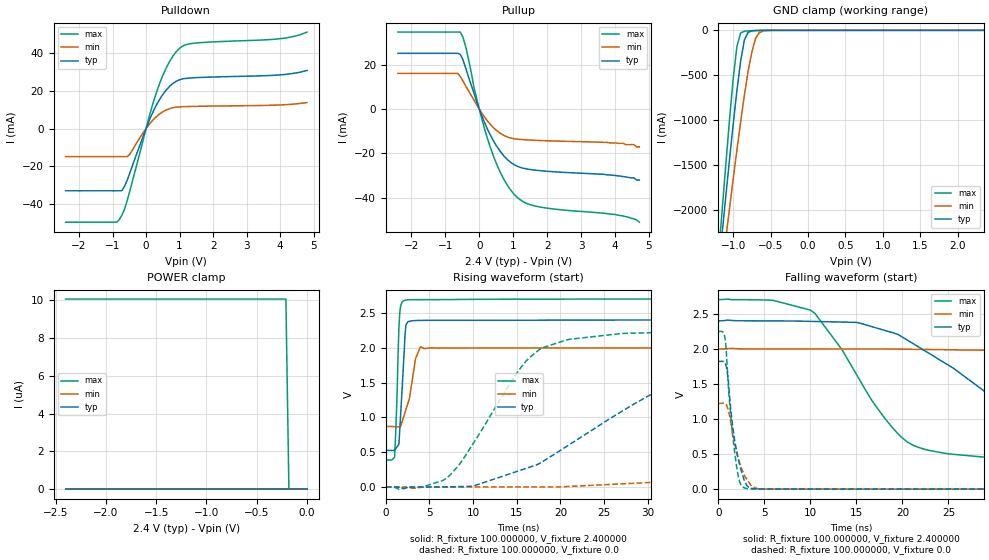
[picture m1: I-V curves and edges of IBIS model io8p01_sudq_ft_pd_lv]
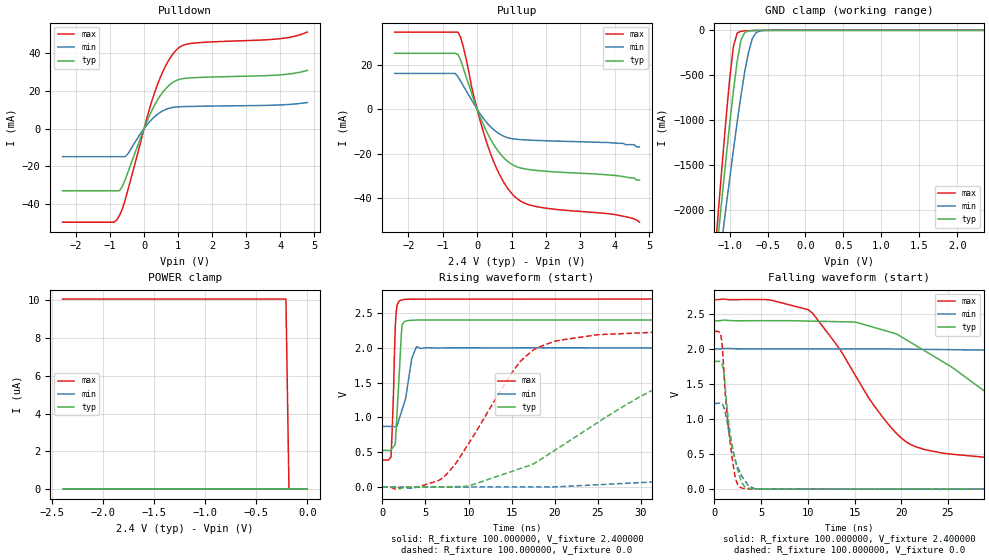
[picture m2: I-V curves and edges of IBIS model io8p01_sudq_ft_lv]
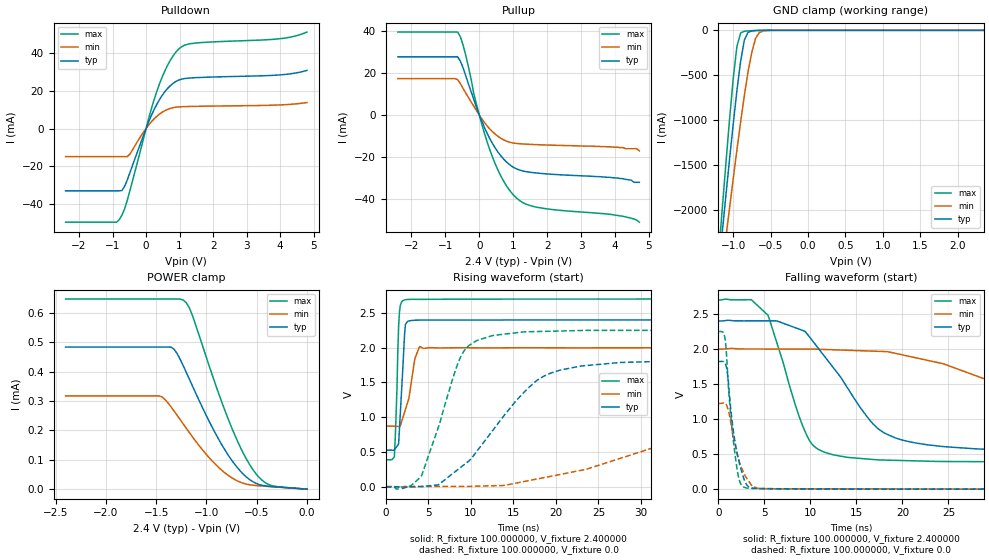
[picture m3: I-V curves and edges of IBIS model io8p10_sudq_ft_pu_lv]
|   stm32f0_444_tssop20 IBIS Model
[IBIS ver]   4.2
[File name]  stm32f0_444_tssop20.ibs
[File Rev]   1.0
[Date]   15-5-2013
[Source] Data Created at STMicroelectronics
[Notes]   File originated from ELDO simulations.
[Disclaimer]  This information is for modeling purpose only and is
   not guaranted. The information is subject to change without
   notice.
[Copyright] Copyright 2015 STMicroelectronics Inc.
[Component] stm32f0_444_tssop20
[Manufacturer] STMicroelectronics
[Package]
| variable   typ   min   max
R_pkg   0.0   NA   NA
L_pkg   0.0H   NA   NA
C_pkg   0.0F   NA   NA
[Pin] signal_name  model_name   R_pin   L_pin   C_pin
1   BOOT0 vpp_test_hv   23.0E-3   1.4E-9   40.0E-15
2   PF0   io8p_sudq_ft   18.1E-3   896.7E-12   15.0E-15
3   PF1   io8p_sudq_ft   16.4E-3   726.7E-12   6.7E-15
4   NRST  ioreset_tc_v33   18.1E-3   896.7E-12   15.0E-15
5   VDDA  POWER   23.0E-3   1.4E-9   40.0E-15
6   PA0   io8p_sudq_ft   23.0E-3   1.4E-9   40.0E-15
7   PA1   io8p_sudq_ft   18.1E-3   896.7E-12   15.0E-15
8   PA2   io8p_sudq_ft   16.4E-3   726.7E-12   6.7E-15
9   PA3   io8p_sudq_ft   18.1E-3   896.7E-12   15.0E-15
10   PA4   io8p_sudq_ft   23.0E-3   1.4E-9   40.0E-15
11   PA5   io8p_sudq_ft   23.0E-3   1.4E-9   40.0E-15
12   PA6   io8p_sudq_ft   18.1E-3   896.7E-12   15.0E-15
13   PA7   io8p_sudq_ft   16.4E-3   726.7E-12   6.7E-15
14   PB1   io8p_sudq_ft   18.1E-3   896.7E-12   15.0E-15
15   VSS   GND   23.0E-3   1.4E-9   40.0E-15
16   VDD   POWER   23.0E-3   1.4E-9   40.0E-15
17   PA9   io8p_sudq_ft   18.1E-3   896.7E-12   15.0E-15
18   PA10  io8p_sudq_ft   16.4E-3   726.7E-12   6.7E-15
19   PA13  io8p_sudq_ft   18.1E-3   896.7E-12   15.0E-15
20   PA14  io8p_sudq_ft   23.0E-3   1.4E-9   40.0E-15
[Model Selector] io8p_sudq_ft
io8p01_sudq_ft_pd_lv  "SPEED01 2P0V, PD=40kOhm"
io8p01_sudq_ft_pu_lv  "SPEED01 2P0V, PU=40kOhm"
io8p01_sudq_ft_lv  "SPEED01 2P0V"
io8p10_sudq_ft_pd_lv  "SPEED10 2P0V, PD=40kOhm"
io8p10_sudq_ft_pu_lv  "SPEED10 2P0V, PU=40kOhm"
io8p10_sudq_ft_lv  "SPEED10 2P0V"
io8p11_sudq_ft_pd_lv  "SPEED11 2P0V, PD=40kOhm"
io8p11_sudq_ft_pu_lv  "SPEED11 2P0V, PU=40kOhm"
io8p11_sudq_ft_lv  "SPEED11 2P0V"
io8p01_sudq_ft_pd  "SPEED01, PD=40kOhm"
io8p01_sudq_ft_pu  "SPEED01, PU=40kOhm"
io8p01_sudq_ft  "SPEED01"
io8p10_sudq_ft_pd  "SPEED10, PD=40kOhm"
io8p10_sudq_ft_pu  "SPEED10, PU=40kOhm"
io8p10_sudq_ft  "SPEED10"
io8p11_sudq_ft_pd  "SPEED11, PD=40kOhm"
io8p11_sudq_ft_pu  "SPEED11, PU=40kOhm"
io8p11_sudq_ft  "SPEED11"
[Model Selector] ioreset_tc_v33
ioreset_tc_v33_pu_lv  "IORESET 2V + PU=40kOhm"
ioreset_tc_v33_nopu_lv  "IORESET 2V"
ioreset_tc_v33_pu  "IORESET + PU=40kOhm"
ioreset_tc_v33_nopu  "IORESET"
[Model Selector] vpp_test_hv
vpp_test_hv_3p3  "Input Buffer"
vpp_test_hv_2p4  "Input Buffer 2P0V"
| Models and submodels in the file (24): io8p01_sudq_ft_pd_lv (I/O), io8p01_sudq_ft_pu_lv (I/O), io8p01_sudq_ft_lv (I/O), io8p10_sudq_ft_pd_lv (I/O), io8p10_sudq_ft_pu_lv (I/O), io8p10_sudq_ft_lv (I/O), io8p11_sudq_ft_pd_lv (I/O), io8p11_sudq_ft_pu_lv (I/O), io8p11_sudq_ft_lv (I/O), io8p01_sudq_ft_pd (I/O), io8p01_sudq_ft_pu (I/O), io8p01_sudq_ft (I/O), io8p10_sudq_ft_pd (I/O), io8p10_sudq_ft_pu (I/O), io8p10_sudq_ft (I/O), io8p11_sudq_ft_pd (I/O), io8p11_sudq_ft_pu (I/O), io8p11_sudq_ft (I/O), ioreset_tc_v33_pu_lv (I/O_open_drain), ioreset_tc_v33_nopu_lv (I/O_open_drain), ioreset_tc_v33_pu (I/O_open_drain), ioreset_tc_v33_nopu (I/O_open_drain), vpp_test_hv_2p4 (Input), vpp_test_hv_3p3 (Input)
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|   Model io8p01_sudq_ft_pd_lv
[Model]  io8p01_sudq_ft_pd_lv
Model_type I/O
Polarity   Non-Inverting
Enable   Active-Low
Vinl =   0.720000V
Vinh =   1.680000V
Vmeas =  1.200000V
Cref =   50.000000pF
Rref =   100.000000M
Vref =   0.0V
C_comp   1.970100pF   1.887900pF   2.069400pF
[Temperature Range]   25.000000   0.125000k   -40.000000
[Pullup Reference]   2.400000V   2.000000V   2.700000V
[Pulldown Reference]   0.0V   0.0V   0.0V
[POWER Clamp Reference]   2.400000V   2.000000V   2.700000V
[GND Clamp Reference]   0.0V   0.0V   0.0V
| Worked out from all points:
|   slope of the pulldown table from 0 to 0.36 V, typ, clamps not added: 25.5 ohm
|   slope of the pullup table from 0 to 0.36 V, typ, clamps not added: 28.4 ohm
|   GND clamp passes 1 mA (typ) near -0.64 V on its own axis
|   rising waveform, R_fixture 100.000000, V_fixture 2.400000: 20-80 % time 499ps typ, 1.06ns min, 336ps max; typ from 0.525 V to 2.4 V
|   rising waveform, R_fixture 100.000000, V_fixture 0.0: 20-80 % time 14.6ns typ, 43.7ns min, 6.88ns max; typ from 0 V to 1.82 V
|   falling waveform, R_fixture 100.000000, V_fixture 2.400000: 20-80 % time 12.9ns typ, 32.5ns min, 7.07ns max; typ from 2.4 V to 0.525 V
|   falling waveform, R_fixture 100.000000, V_fixture 0.0: 20-80 % time 1.15ns typ, 1.36ns min, 910ps max; typ from 1.82 V to 0 V
[Pulldown]
|Voltage   I(typ)   I(min)   I(max)
-2.4V     -33.16mA   -14.98mA   -49.86mA
-880mV    -33.16mA   -14.98mA   -49.86mA
-800mV    -33.16mA   -14.98mA   -48.55mA
-640mV    -30.75mA   -14.98mA   -42.76mA
-480mV    -23.43mA   -13.57mA   -32.92mA
80mV      3.651mA    1.905mA    5.506mA
400mV     15.37mA    7.665mA    23.73mA
720mV     22.75mA    10.69mA    36.23mA
1.04V     26.18mA    11.57mA    43.27mA
1.52V     27.09mA    11.81mA    45.55mA
4V        28.55mA    12.55mA    47.81mA
4.8V      30.9mA     13.81mA    51.31mA
[Pullup]
|Voltage   I(typ)   I(min)   I(max)
-2.4V     25.2mA     16.13mA    34.79mA
-640mV    25.2mA     16.13mA    34.79mA
-560mV    24.71mA    14.75mA    34.79mA
-400mV    18.51mA    10.48mA    28.09mA
-160mV    7.338mA    4.152mA    10.02mA
80mV      -3.229mA   -1.94mA    -4.736mA
400mV     -13.82mA   -8.081mA   -20.45mA
800mV     -22.31mA   -12.38mA   -33.66mA
1.2V      -26.24mA   -13.65mA   -40.83mA
1.76V     -27.69mA   -14.12mA   -44.07mA
4V        -29.9mA    -15.2mA    -47.5mA
4.72V     -32mA      -17mA      -51mA
[GND_clamp]
|Voltage   I(typ)   I(min)   I(max)
-2.4V     -9.788A    -9.782A    -9.734A
-1.2V     -2.718A    -3.021A    -2.568A
-1.15V    -2.29A     -2.675A    -2.036A
-1.1V     -1.868A    -2.333A    -1.515A
-1.05V    -1.454A    -1.995A    -1.012A
-950mV    -674.5mA   -1.337A    -180.6mA
-900mV    -345.2mA   -1.023A    -29.74mA
-850mV    -106.4mA   -726mA     -10.14mA
-750mV    -6.411mA   -244mA     -4.042mA
-700mV    -2.572mA   -88.62mA   -2.346mA
-600mV    -429.6uA   -7.75mA    -383.5uA
2.35V     59.77uA    46.33uA    66.89uA
[POWER_clamp]
|Voltage   I(typ)   I(min)   I(max)
-2.4V     0A         0A         10.06uA
-210mV    0A         0A         10.06uA
-180mV    0A         0A         0A
0V        0A         0A         0A
[Ramp]
| variable   typ   min   max
dV/dt_r  1.09218/14.55718n   0.73266/43.64565n   1.34874/6.87247n
dV/dt_f  1.12429/12.86053n   0.67801/32.45722n   1.38701/7.06387n
R_load = 100.000000
[Rising Waveform]
R_fixture= 100.000000
V_fixture= 2.400000
V_fixture_min= 2.000000
V_fixture_max= 2.700000
|time   V(typ)   V(min)   V(max)
0s        524.8mV    868.7mV    387.2mV
1.001ns   533mV      867mV      427.7mV
1.301ns   579.7mV    865.4mV    1.395V
1.502ns   618.4mV    864.7mV    2.307V
1.602ns   837.8mV    864.4mV    2.512V
2.102ns   1.961V     1.034V     2.677V
2.302ns   2.331V     1.113V     2.684V
3.403ns   2.39V      1.843V     2.691V
4.004ns   2.392V     2.014V     2.691V
49.85ns   2.399V     1.999V     2.699V
[Rising Waveform]
R_fixture= 100.000000
V_fixture= 0.0
V_fixture_min= 0.0
V_fixture_max= 0.0
|time   V(typ)   V(min)   V(max)
0s        1.768nV    15.89nV    1.355nV
7.007ns   1.867mV    822uV      130.1mV
15.02ns   222.8mV    610.6uV    1.635V
17.52ns   330.7mV    351.7uV    1.966V
27.03ns   1.085V     44.44mV    2.204V
34.53ns   1.55V      90.81mV    2.229V
43.04ns   1.723V     239mV      2.246V
84.08ns   1.82V      945.5mV    2.248V
103.1ns   1.82V      1.111V     2.248V
249.2ns   1.82V      1.221V     2.248V
[Falling Waveform]
R_fixture= 100.000000
V_fixture= 2.400000
V_fixture_min= 2.000000
V_fixture_max= 2.700000
|time   V(typ)   V(min)   V(max)
0s        2.399V     1.999V     2.699V
10.01ns   2.391V     1.998V     2.551V
15.02ns   2.376V     1.997V     1.633V
20.02ns   2.165V     1.994V     725.2mV
29.53ns   1.332V     1.979V     449.6mV
35.04ns   877.6mV    1.964V     425.1mV
42.54ns   673.2mV    1.851V     405.8mV
67.07ns   552.7mV    1.286V     389.2mV
85.59ns   536.1mV    1.035V     387.2mV
249.2ns   524.8mV    868.7mV    387.2mV
[Falling Waveform]
R_fixture= 100.000000
V_fixture= 0.0
V_fixture_min= 0.0
V_fixture_max= 0.0
|time   V(typ)   V(min)   V(max)
0s        1.82V      1.221V     2.248V
700.7ps   1.801V     1.221V     2.178V
800.8ps   1.783V     1.214V     2.095V
1.001ns   1.652V     1.164V     1.701V
1.401ns   1.088V     921.6mV    989mV
1.802ns   687.3mV    646.2mV    513.2mV
2.302ns   364.2mV    381.5mV    115.5mV
2.903ns   104.2mV    178.7mV    14.94mV
4.705ns   1.559mV    3.204mV    789.6uV
49.85ns   1.768nV    15.89nV    1.355nV
|   Model io8p01_sudq_ft_lv
[Model]  io8p01_sudq_ft_lv
Model_type I/O
Polarity   Non-Inverting
Enable   Active-Low
Vinl =   0.720000V
Vinh =   1.680000V
Vmeas =  1.200000V
Cref =   50.000000pF
Rref =   100.000000M
Vref =   0.0V
C_comp   1.970100pF   1.887900pF   2.069400pF
[Temperature Range]   25.000000   0.125000k   -40.000000
[Pullup Reference]   2.400000V   2.000000V   2.700000V
[Pulldown Reference]   0.0V   0.0V   0.0V
[POWER Clamp Reference]   2.400000V   2.000000V   2.700000V
[GND Clamp Reference]   0.0V   0.0V   0.0V
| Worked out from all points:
|   slope of the pulldown table from 0 to 0.36 V, typ, clamps not added: 25.5 ohm
|   slope of the pullup table from 0 to 0.36 V, typ, clamps not added: 28.4 ohm
|   GND clamp passes 1 mA (typ) near -0.64 V on its own axis
|   rising waveform, R_fixture 100.000000, V_fixture 2.400000: 20-80 % time 499ps typ, 1.06ns min, 336ps max; typ from 0.525 V to 2.4 V
|   rising waveform, R_fixture 100.000000, V_fixture 0.0: 20-80 % time 14.5ns typ, 43.7ns min, 6.87ns max; typ from 0 V to 1.82 V
|   falling waveform, R_fixture 100.000000, V_fixture 2.400000: 20-80 % time 13ns typ, 32.3ns min, 7.05ns max; typ from 2.4 V to 0.525 V
|   falling waveform, R_fixture 100.000000, V_fixture 0.0: 20-80 % time 1.16ns typ, 1.39ns min, 931ps max; typ from 1.82 V to 0 V
[Pulldown]
|Voltage   I(typ)   I(min)   I(max)
-2.4V     -33.16mA   -14.98mA   -49.86mA
-880mV    -33.16mA   -14.98mA   -49.86mA
-800mV    -33.16mA   -14.98mA   -48.55mA
-640mV    -30.75mA   -14.98mA   -42.76mA
-480mV    -23.43mA   -13.57mA   -32.92mA
80mV      3.651mA    1.905mA    5.506mA
400mV     15.37mA    7.665mA    23.73mA
720mV     22.75mA    10.69mA    36.23mA
1.04V     26.18mA    11.57mA    43.27mA
1.52V     27.09mA    11.81mA    45.55mA
4V        28.55mA    12.55mA    47.81mA
4.8V      30.9mA     13.81mA    51.31mA
[Pullup]
|Voltage   I(typ)   I(min)   I(max)
-2.4V     25.21mA    16.13mA    34.79mA
-640mV    25.21mA    16.13mA    34.79mA
-560mV    24.72mA    14.75mA    34.79mA
-400mV    18.51mA    10.48mA    28.09mA
-160mV    7.322mA    4.15mA     10.02mA
80mV      -3.229mA   -1.94mA    -4.736mA
400mV     -13.82mA   -8.081mA   -20.45mA
800mV     -22.31mA   -12.38mA   -33.66mA
1.2V      -26.24mA   -13.65mA   -40.83mA
1.76V     -27.69mA   -14.12mA   -44.07mA
4V        -29.9mA    -15.2mA    -47.5mA
4.72V     -32mA      -17mA      -51mA
[GND_clamp]
|Voltage   I(typ)   I(min)   I(max)
-2.4V     -9.788A    -9.782A    -9.734A
-1.2V     -2.718A    -3.02A     -2.568A
-1.15V    -2.29A     -2.675A    -2.036A
-1.1V     -1.868A    -2.333A    -1.515A
-1.05V    -1.454A    -1.995A    -1.012A
-950mV    -674.5mA   -1.337A    -180.5mA
-900mV    -345.2mA   -1.023A    -29.72mA
-850mV    -106.4mA   -726mA     -10.13mA
-750mV    -6.396mA   -244mA     -4.026mA
-700mV    -2.558mA   -88.61mA   -2.329mA
-600mV    -416uA     -7.739mA   -368uA
2.35V     0A         0A         0A
[POWER_clamp]
|Voltage   I(typ)   I(min)   I(max)
-2.4V     0A         0A         10.06uA
-210mV    0A         0A         10.06uA
-180mV    0A         0A         0A
0V        0A         0A         0A
[Ramp]
| variable   typ   min   max
dV/dt_r  1.09308/14.53591n   0.73368/43.60005n   1.34946/6.86189n
dV/dt_f  1.12469/12.94342n   0.67781/32.23620n   1.38756/7.04174n
R_load = 100.000000
[Rising Waveform]
R_fixture= 100.000000
V_fixture= 2.400000
V_fixture_min= 2.000000
V_fixture_max= 2.700000
|time   V(typ)   V(min)   V(max)
0s        525.2mV    870.3mV    387.4mV
1.001ns   533.4mV    868.6mV    427.9mV
1.301ns   580.2mV    867mV      1.396V
1.502ns   618.9mV    866.4mV    2.308V
1.702ns   1.058V     877.1mV    2.607V
2.202ns   2.2V       1.075V     2.686V
2.703ns   2.383V     1.274V     2.696V
3.403ns   2.395V     1.844V     2.698V
4.004ns   2.398V     2.016V     2.698V
49.85ns   2.4V       2V         2.7V
[Rising Waveform]
R_fixture= 100.000000
V_fixture= 0.0
V_fixture_min= 0.0
V_fixture_max= 0.0
|time   V(typ)   V(min)   V(max)
0s        1.81nV     16.19nV    1.388nV
7.007ns   1.867mV    817.4uV    130.2mV
16.52ns   286.2mV    456uV      1.866V
20.02ns   528mV      1.164mV    2.095V
25.03ns   931.2mV    32.13mV    2.189V
37.04ns   1.629V     132.6mV    2.24V
54.55ns   1.791V     444.2mV    2.251V
84.08ns   1.821V     947.3mV    2.249V
106.1ns   1.822V     1.128V     2.249V
249.2ns   1.822V     1.223V     2.249V
[Falling Waveform]
R_fixture= 100.000000
V_fixture= 2.400000
V_fixture_min= 2.000000
V_fixture_max= 2.700000
|time   V(typ)   V(min)   V(max)
0s        2.4V       2V         2.7V
10.01ns   2.397V     2V         2.56V
15.02ns   2.383V     2V         1.637V
20.02ns   2.171V     1.997V     726.6mV
29.03ns   1.387V     1.983V     453.9mV
37.04ns   789.8mV    1.94V      415.8mV
52.55ns   592.4mV    1.669V     394.5mV
72.57ns   546.2mV    1.209V     388.6mV
99.1ns    528mV      969.1mV    387.4mV
249.2ns   525.2mV    870.3mV    387.4mV
[Falling Waveform]
R_fixture= 100.000000
V_fixture= 0.0
V_fixture_min= 0.0
V_fixture_max= 0.0
|time   V(typ)   V(min)   V(max)
0s        1.822V     1.223V     2.249V
700.7ps   1.802V     1.223V     2.18V
800.8ps   1.785V     1.216V     2.097V
1.001ns   1.655V     1.166V     1.704V
1.201ns   1.378V     1.071V     1.289V
1.902ns   616.6mV    591.6mV    436.6mV
2.302ns   369.3mV    388.2mV    131.7mV
2.903ns   108.1mV    191.2mV    18.1mV
4.705ns   2.197mV    4.103mV    1.139mV
49.85ns   1.81nV     16.19nV    1.388nV
|   Model io8p10_sudq_ft_pu_lv
[Model]  io8p10_sudq_ft_pu_lv
Model_type I/O
Polarity   Non-Inverting
Enable   Active-Low
Vinl =   0.720000V
Vinh =   1.680000V
Vmeas =  1.200000V
Cref =   50.000000pF
Rref =   100.000000M
Vref =   0.0V
C_comp   1.970100pF   1.887900pF   2.069400pF
[Temperature Range]   25.000000   0.125000k   -40.000000
[Pullup Reference]   2.400000V   2.000000V   2.700000V
[Pulldown Reference]   0.0V   0.0V   0.0V
[POWER Clamp Reference]   2.400000V   2.000000V   2.700000V
[GND Clamp Reference]   0.0V   0.0V   0.0V
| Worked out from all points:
|   slope of the pulldown table from 0 to 0.36 V, typ, clamps not added: 25.5 ohm
|   slope of the pullup table from 0 to 0.36 V, typ, clamps not added: 28.4 ohm
|   GND clamp passes 1 mA (typ) near -0.64 V on its own axis
|   rising waveform, R_fixture 100.000000, V_fixture 2.400000: 20-80 % time 500ps typ, 1.06ns min, 335ps max; typ from 0.527 V to 2.4 V
|   rising waveform, R_fixture 100.000000, V_fixture 0.0: 20-80 % time 7.39ns typ, 21.1ns min, 3.53ns max; typ from 0.001 V to 1.82 V
|   falling waveform, R_fixture 100.000000, V_fixture 2.400000: 20-80 % time 6.28ns typ, 17.7ns min, 3.33ns max; typ from 2.4 V to 0.527 V
|   falling waveform, R_fixture 100.000000, V_fixture 0.0: 20-80 % time 1.16ns typ, 1.4ns min, 916ps max; typ from 1.82 V to 0.001 V
[Pulldown]
|Voltage   I(typ)   I(min)   I(max)
-2.4V     -33.16mA   -14.98mA   -49.86mA
-880mV    -33.16mA   -14.98mA   -49.86mA
-800mV    -33.16mA   -14.98mA   -48.55mA
-640mV    -30.75mA   -14.98mA   -42.77mA
-480mV    -23.43mA   -13.57mA   -32.92mA
80mV      3.651mA    1.905mA    5.506mA
400mV     15.37mA    7.665mA    23.73mA
720mV     22.75mA    10.69mA    36.23mA
1.04V     26.18mA    11.57mA    43.27mA
1.52V     27.09mA    11.81mA    45.55mA
4V        28.55mA    12.55mA    47.81mA
4.8V      30.9mA     13.81mA    51.31mA
[Pullup]
|Voltage   I(typ)   I(min)   I(max)
-2.4V     27.74mA    17.38mA    39.53mA
-640mV    27.74mA    16.88mA    39.53mA
-560mV    25.73mA    15.04mA    37.34mA
-480mV    22.58mA    12.74mA    33.42mA
-80mV     3.427mA    2.071mA    4.957mA
160mV     -6.219mA   -3.715mA   -9.137mA
320mV     -11.51mA   -6.781mA   -16.98mA
720mV     -21mA      -11.8mA    -31.53mA
1.12V     -25.77mA   -13.54mA   -39.82mA
1.76V     -27.69mA   -14.12mA   -44.07mA
3.84V     -29.6mA    -15.1mA    -47.2mA
4.72V     -32mA      -17mA      -51mA
[GND_clamp]
|Voltage   I(typ)   I(min)   I(max)
-2.4V     -9.788A    -9.782A    -9.734A
-1.2V     -2.718A    -3.02A     -2.568A
-1.15V    -2.29A     -2.675A    -2.036A
-1.1V     -1.868A    -2.333A    -1.515A
-1.05V    -1.454A    -1.995A    -1.012A
-950mV    -674.5mA   -1.337A    -180.5mA
-900mV    -345.2mA   -1.023A    -29.72mA
-850mV    -106.4mA   -726mA     -10.13mA
-750mV    -6.396mA   -244mA     -4.026mA
-700mV    -2.558mA   -88.61mA   -2.329mA
-600mV    -416uA     -7.739mA   -368uA
2.35V     0A         0A         0A
[POWER_clamp]
|Voltage   I(typ)   I(min)   I(max)
-2.4V     483.8uA    317.4uA    647uA
-1.47V    483.8uA    317.4uA    647uA
-1.32V    475.6uA    265.2uA    647uA
-1.23V    419.7uA    221.6uA    643.3uA
-1.17V    374.8uA    192.7uA    617.6uA
-1.14V    352.1uA    178.7uA    591.9uA
-840mV    147uA      62.15uA    289.6uA
-690mV    72.24uA    27.76uA    162.7uA
-540mV    25.74uA    13.55uA    67.63uA
-450mV    13.38uA    10.75uA    31.36uA
-360mV    9.231uA    8.535uA    12.97uA
0V        0A         0A         0A
[Ramp]
| variable   typ   min   max
dV/dt_r  1.09257/7.38126n   0.73299/21.13981n   1.34920/3.52606n
dV/dt_f  1.12405/6.26972n   0.67519/17.74591n   1.38687/3.32829n
R_load = 100.000000
[Rising Waveform]
R_fixture= 100.000000
V_fixture= 2.400000
V_fixture_min= 2.000000
V_fixture_max= 2.700000
|time   V(typ)   V(min)   V(max)
0s        526.5mV    872.5mV    388.6mV
1.001ns   534.6mV    870.8mV    428.2mV
1.301ns   580.6mV    869.2mV    1.393V
1.502ns   618.8mV    868.6mV    2.312V
1.702ns   1.058V     879.1mV    2.61V
2.102ns   1.96V      1.035V     2.683V
2.302ns   2.337V     1.113V     2.69V
3.403ns   2.395V     1.84V      2.696V
4.004ns   2.398V     2.018V     2.696V
49.85ns   2.4V       2V         2.7V
[Rising Waveform]
R_fixture= 100.000000
V_fixture= 0.0
V_fixture_min= 0.0
V_fixture_max= 0.0
|time   V(typ)   V(min)   V(max)
0s        1.057mV    1.357mV    941.6uV
2.803ns   2.743mV    -4.311mV   6.043mV
4.204ns   4.237mV    2.829mV    160mV
6.206ns   30.25mV    4.308mV    867.3mV
8.809ns   280mV      4.087mV    1.872V
12.61ns   817.4mV    14.56mV    2.176V
17.82ns   1.535V     112.7mV    2.233V
23.02ns   1.737V     237.9mV    2.248V
49.25ns   1.822V     1.075V     2.25V
99.7ns    1.822V     1.224V     2.25V
[Falling Waveform]
R_fixture= 100.000000
V_fixture= 2.400000
V_fixture_min= 2.000000
V_fixture_max= 2.700000
|time   V(typ)   V(min)   V(max)
0s        2.4V       2V         2.7V
3.604ns   2.401V     2V         2.702V
5.405ns   2.402V     2V         2.482V
9.61ns    2.224V     2V         771.1mV
12.61ns   1.714V     1.989V     487.5mV
17.42ns   856.8mV    1.967V     418.1mV
24.42ns   608.6mV    1.79V      395.7mV
43.84ns   535.4mV    1.055V     388.6mV
52.45ns   528.4mV    947.9mV    388.6mV
99.7ns    526.5mV    872.5mV    388.6mV
[Falling Waveform]
R_fixture= 100.000000
V_fixture= 0.0
V_fixture_min= 0.0
V_fixture_max= 0.0
|time   V(typ)   V(min)   V(max)
0s        1.822V     1.224V     2.25V
700.7ps   1.803V     1.224V     2.181V
800.8ps   1.785V     1.216V     2.099V
1.001ns   1.656V     1.167V     1.707V
1.401ns   1.093V     925.2mV    997.9mV
1.902ns   618.4mV    593.3mV    424.7mV
2.302ns   371.4mV    390.6mV    125.2mV
2.903ns   111.3mV    194.4mV    23.9mV
4.705ns   8.256mV    8.438mV    9.524mV
49.85ns   1.057mV    1.357mV    941.6uV
